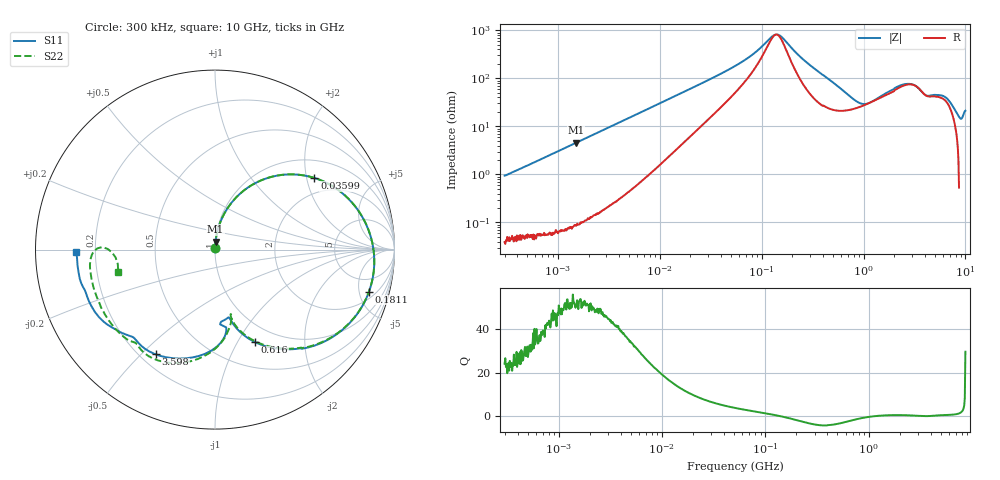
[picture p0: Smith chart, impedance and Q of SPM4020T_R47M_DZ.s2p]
! S-Parameter Data Generated by TDK Corporation
! Copyright(C) 2024 TDK Corporation.
! All Rights Reserved.
! TDK P/N: SPM4020T-R47M-DZ (SMD / SMT Inductor (Coil))
! Property: L=470nH at 100kHz
! Size(LxWxT): 4.3x4.1x2mm
! Model Type: s2p (Touchstone File Format Version 1.0)
! Frequency: DC=Yes Start=0.3MHz Stop=10000MHz 802points Log-sweep
! Model Generated on May 28, 2024
! Terms and conditions regarding TDK Simulation Models:
! 1)This simulation model is being provided solely for informational
!  purposes. Please refer to the specifications of the products in
!  terms of detailed characteristics of such products.
! 2)In no event shall TDK Corporation of any of its subsidiaries be
!  liable for any loss or damage arising, directly or indirectly,
!  from any information contained in this simulation model, including,
!  but not limited to loss or damages arising from any inaccuracies,
!  omissions or errors in connection with such information.
! 3)Any and all copyrights on this simulation model are owned by
!  TDK Corporation.  Duplication or redistribution of this simulation
!  model without prior written permission from TDK Corporation
!  is prohibited.
! 4)This simulation model is subject to any modification or change
!  without any prior notice.
! 5)Neither TDK Corporation nor any of its subsidiaries shall make any
!  warranty, express or implied, including but not limited to the
!  correctness, implied warranties of merchantability and fitness for
!  a particular purpose with respect to this simulation models.
! 6)The use of this simulation model shall be deemed to have consented
!  to the terms and conditions hereof.
! Port Assignments:
!  1 ---@@@--- 2
! Applicable Conditions:
!  Temperature = 25 degC
!  DC Bias Current = 0 A
!  Small Signal Operation
# Hz S MA R 50
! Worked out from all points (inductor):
!   801 points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, 300 kHz to 10 GHz, reference 50 ohm
!   read as one part in series: L = 489 nH near 318.3 kHz
!   highest Q = 52.6 at 1.507 MHz (marker M1), where L = 481 nH
!   self-resonance near 138.8 MHz
!   S11 on the Smith chart (normalised r, x): 300 kHz: 1.00, +0.02; 35.99 MHz: 1.49, +2.23; 181.1 MHz: 2.79, -6.25; 616 MHz: 0.79, -1.19; 3.598 GHz: 0.26, -0.55; 10 GHz: 0.13, -0.01
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300000  0.009803 88.2  0.9993 -0.5  0.9992 -0.5  0.009928 90.1
1507188  0.04514 86.3  0.9981 -2.6  0.998 -2.6  0.04513 86.4
1713600  0.05124 86.0  0.9975 -3.0  0.9977 -3.0  0.05124 86.1
9671944  0.2737 70.8  0.9478 -16.3  0.9481 -16.2  0.2736 70.8
2.063197e7  0.5039 53.0  0.8117 -30.9  0.812 -30.9  0.5038 53.0
3.598933e7  0.6827 35.8  0.6161 -43.6  0.6162 -43.6  0.6827 35.8
5.477226e7  0.7844 22.6  0.4387 -51.1  0.4388 -51.1  0.7843 22.7
8.27046e7  0.8504 10.3  0.2666 -52.7  0.2667 -52.7  0.8504 10.4
1.340254e8  0.8904 -4.7  0.1106 -13.1  0.1106 -13.1  0.8903 -4.5
1.518127e8  0.8929 -8.9  0.1148 13.9  0.1148 13.9  0.8928 -8.7
1.810762e8  0.8895 -15.3  0.1671 37.6  0.1672 37.6  0.8894 -15.0
3.126428e8  0.8087 -38.0  0.4311 39.1  0.4311 39.1  0.8082 -37.6
4.388767e8  0.6976 -52.8  0.5814 25.4  0.5815 25.4  0.6962 -52.5
6.15965e8  0.5616 -66.6  0.686 8.1  0.6861 8.1  0.5584 -66.3
9.903836e8  0.4098 -77.1  0.7149 -18.6  0.7151 -18.6  0.3982 -76.5
1.767019e9  0.4008 -84.5  0.5631 -52.9  0.5633 -52.9  0.4203 -77.9
2.38587e9  0.5244 -87.0  0.4449 -67.3  0.4451 -67.3  0.5408 -88.6
3.598403e9  0.6701 -119.5  0.3291 -75.2  0.3292 -75.3  0.6976 -119.3
6.333834e9  0.7282 -144.7  0.2558 -117.5  0.2558 -117.5  0.7091 -142.0
8.211115e9  0.76 -162.9  0.1909 -145.3  0.1908 -145.4  0.7059 -168.4
9.217363e9  0.7707 -170.8  0.1488 -158.3  0.1491 -158.2  0.6562 179.5
1e10  0.7719 -179.0  0.123 -155.3  0.123 -155.5  0.5534 -167.0
